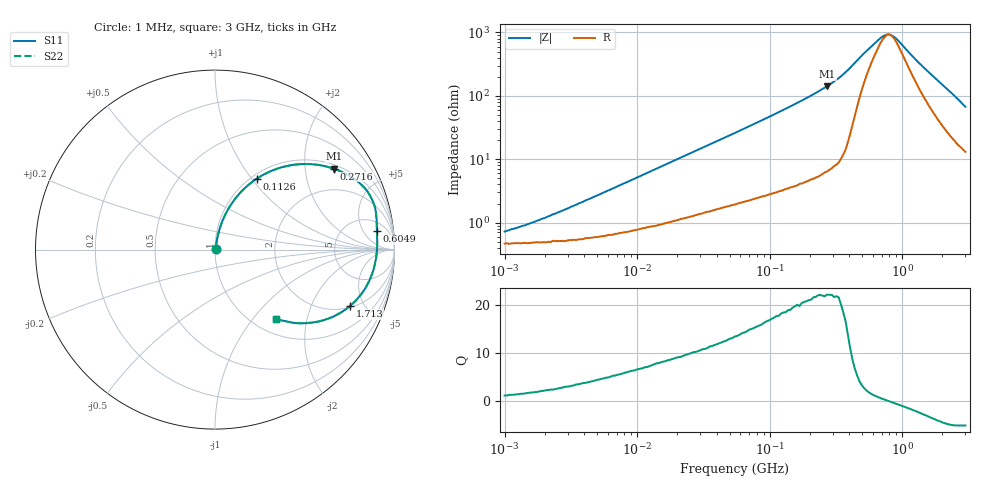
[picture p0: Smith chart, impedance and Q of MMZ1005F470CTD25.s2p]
! S-Parameter Data Generated by TDK Corporation
! Copyright(C) 2025 TDK Corporation.
! All Rights Reserved.
! TDK P/N: MMZ1005F470CTD25 (Chip Bead)
! Property: |Z|=47ohm at 100MHz
! Size(LxWxT): 1x0.5x0.5mm
! Model Type: s2p (Touchstone File Format Version 1.0)
! Frequency: DC=Yes Start=1MHz Stop=3000MHz 202points Log-sweep
! Model Generated on Feb. 6, 2025
! Terms and conditions regarding TDK Simulation Models:
! 1)This simulation model is being provided solely for informational
!  purposes. Please refer to the specifications of the products in
!  terms of detailed characteristics of such products.
! 2)In no event shall TDK Corporation of any of its subsidiaries be
!  liable for any loss or damage arising, directly or indirectly,
!  from any information contained in this simulation model, including,
!  but not limited to loss or damages arising from any inaccuracies,
!  omissions or errors in connection with such information.
! 3)Any and all copyrights on this simulation model are owned by
!  TDK Corporation.  Duplication or redistribution of this simulation
!  model without prior written permission from TDK Corporation
!  is prohibited.
! 4)This simulation model is subject to any modification or change
!  without any prior notice.
! 5)Neither TDK Corporation nor any of its subsidiaries shall make any
!  warranty, express or implied, including but not limited to the
!  correctness, implied warranties of merchantability and fitness for
!  a particular purpose with respect to this simulation models.
! 6)The use of this simulation model shall be deemed to have consented
!  to the terms and conditions hereof.
! Port Assignments:
!  1 ---@@@--- 2
! Applicable Conditions:
!  Temperature = 25 degC
!  DC Bias Current = 0 A
!  Small Signal Operation
# Hz S MA R 50
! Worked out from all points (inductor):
!   201 points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, 1 MHz to 3 GHz, reference 50 ohm
!   read as one part in series: L = 84.6 nH near 2.947 MHz
!   highest Q = 22 at 271.6 MHz (marker M1), where L = 83.3 nH
!   self-resonance near 798.6 MHz
!   S11 on the Smith chart (normalised r, x): 1 MHz: 1.01, +0.01; 112.6 MHz: 1.06, +1.06; 271.6 MHz: 1.13, +2.84; 604.9 MHz: 9, +10; 1.713 GHz: 2.10, -3.92; 3 GHz: 1.26, -1.32
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1000000  0.0072 49.6  0.9953 -0.3  0.9953 -0.3  0.0072 49.6
2055611  0.01201 65.6  0.9951 -0.6  0.9951 -0.6  0.01201 65.6
3900413  0.02122 74.0  0.9944 -1.2  0.9944 -1.2  0.02122 74.0
1.461624e7  0.07288 78.7  0.9882 -4.1  0.9882 -4.1  0.07288 78.7
2.886629e7  0.1375 76.6  0.9774 -7.9  0.9774 -7.9  0.1375 76.6
5.477226e7  0.2475 71.4  0.9507 -14.3  0.9507 -14.3  0.2475 71.4
8.173662e7  0.3522 65.8  0.9137 -20.6  0.9137 -20.6  0.3522 65.8
1.125904e8  0.4586 59.5  0.8631 -27.2  0.8631 -27.2  0.4586 59.5
1.614254e8  0.5974 50.5  0.7727 -36.6  0.7727 -36.6  0.5974 50.5
2.136344e8  0.7101 42.2  0.6719 -45.2  0.6719 -45.2  0.7101 42.2
2.716345e8  0.8013 34.2  0.5632 -53.2  0.5632 -53.2  0.8013 34.2
3.453811e8  0.8805 25.6  0.4321 -61.6  0.4321 -61.6  0.8805 25.6
4.219165e8  0.9188 17.5  0.3028 -65.9  0.3028 -65.9  0.9188 17.5
6.049187e8  0.908 6.5  0.1413 -46.2  0.1413 -46.2  0.908 6.5
7.099691e8  0.905 2.7  0.1053 -24.2  0.1053 -24.2  0.905 2.7
8.005644e8  0.9027 -0.1  0.09728 0.5  0.09728 0.5  0.9027 -0.1
9.0272e8  0.899 -3.0  0.1124 24.5  0.1124 24.5  0.899 -3.0
1.243477e9  0.8762 -11.6  0.2262 51.2  0.2262 51.2  0.8762 -11.6
1.712864e9  0.815 -22.7  0.4002 51.7  0.4002 51.7  0.815 -22.7
2.01032e9  0.758 -29.5  0.5047 47.6  0.5047 47.6  0.758 -29.5
2.359433e9  0.677 -36.9  0.613 41.6  0.613 41.6  0.677 -36.9
3e9  0.5139 -48.5  0.7638 30.3  0.7638 30.3  0.5139 -48.5
